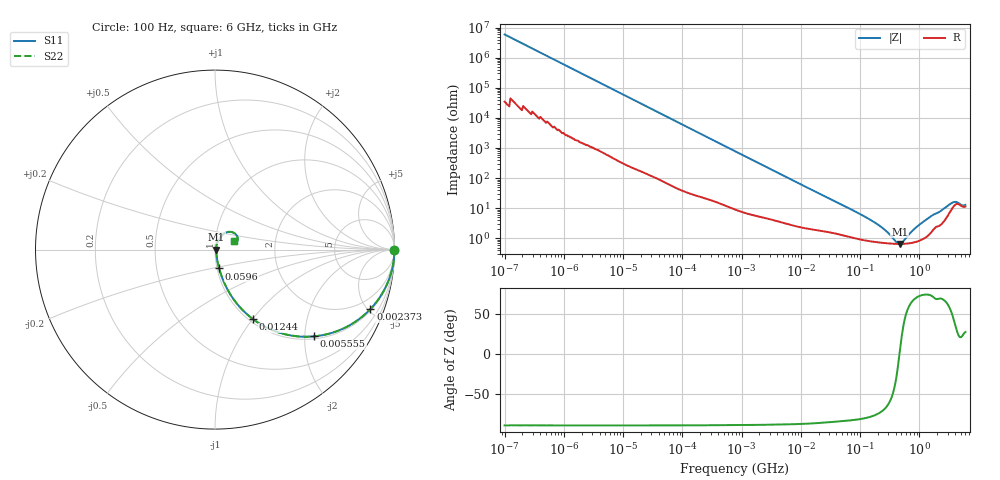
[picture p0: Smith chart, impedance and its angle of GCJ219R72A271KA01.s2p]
!Murata Part Number: GCJ219R72A271KA01
!These Parameters are Measured in Series Mode Connection
!Data Generated on Mar 13, 2026
!  o--ll--o
!Port1  Port2
!  o------o
!Operation Temp=25[degC], DC Bias Voltage=0[V]
!Freq. Start=100[Hz] Stop=6[GHz] 401[Steps]
# Hz S RI R 50
!Freq.(Hz) S11(Real) S11(Imag) S21(Real) S21(Imag) S12(Real) S12(Imag) S22(Real) S22(Imag)
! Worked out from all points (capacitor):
!   401 points, 100 Hz to 6 GHz, reference 50 ohm
!   read as one part in series: C = 270 pF near 109 Hz
!   lowest |Z| = 661 mohm at 467.5 MHz (marker M1)
!   series resonance near 462.7 MHz, so ESL is about 440 pH
!   S11 on the Smith chart (normalised r, x): 100 Hz: open; 2.373 MHz: 1.10, -5.17; 5.555 MHz: 1.06, -2.23; 12.44 MHz: 1.04, -1.01; 59.6 MHz: 1.02, -0.22; 6 GHz: 1.23, +0.12
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100  1 -1.7e-05  1e-07 1.7e-05  1e-07 1.7e-05  1 -1.7e-05
573  1 -9.66e-05  6e-07 9.66e-05  6e-07 9.66e-05  1 -9.66e-05
2008  1 -0.000337  1.8e-06 0.000337  1.8e-06 0.000337  1 -0.000337
40335  0.9999 -0.00671  8.57e-05 0.00671  8.57e-05 0.00671  0.9999 -0.00671
241822  0.9981 -0.0399  0.00194 0.0399  0.00194 0.0399  0.9981 -0.0399
774597  0.9827 -0.1247  0.0173 0.1247  0.0173 0.1247  0.9827 -0.1247
2372521  0.8654 -0.332  0.1346 0.332  0.1346 0.332  0.8654 -0.332
5554849  0.5533 -0.4833  0.4467 0.4833  0.4467 0.4833  0.5533 -0.4833
1.243624e7  0.2122 -0.3881  0.7878 0.3881  0.7878 0.3881  0.2122 -0.3881
1.555665e7  0.1523 -0.3355  0.8477 0.3355  0.8477 0.3355  0.1523 -0.3355
2.662322e7  0.0678 -0.2186  0.9322 0.2186  0.9322 0.2186  0.0678 -0.2186
5.960426e7  0.023 -0.1049  0.977 0.1049  0.977 0.1049  0.023 -0.1049
1.745687e8  0.00875 -0.0331  0.9912 0.0331  0.9912 0.0331  0.00875 -0.0331
3.124326e8  0.00692 -0.012  0.9931 0.012  0.9931 0.012  0.00692 -0.012
4.087225e8  0.0066 -0.00375  0.9934 0.00375  0.9934 0.00375  0.0066 -0.00375
4.674818e8  0.00656 0.000314  0.9934 -0.000314  0.9934 -0.000314  0.00656 0.000314
5.346885e8  0.00661 0.00444  0.9934 -0.00444  0.9934 -0.00444  0.00661 0.00444
7.650043e8  0.00742 0.0163  0.9926 -0.0163  0.9926 -0.0163  0.00742 0.0163
1.046602e9  0.00947 0.0288  0.9905 -0.0288  0.9905 -0.0288  0.00947 0.0288
3.205649e9  0.0747 0.0986  0.9253 -0.0986  0.9253 -0.0986  0.0747 0.0986
4.009986e9  0.1222 0.0775  0.8778 -0.0775  0.8778 -0.0775  0.1222 0.0775
6e9  0.1059 0.0484  0.8941 -0.0484  0.8941 -0.0484  0.1059 0.0484
